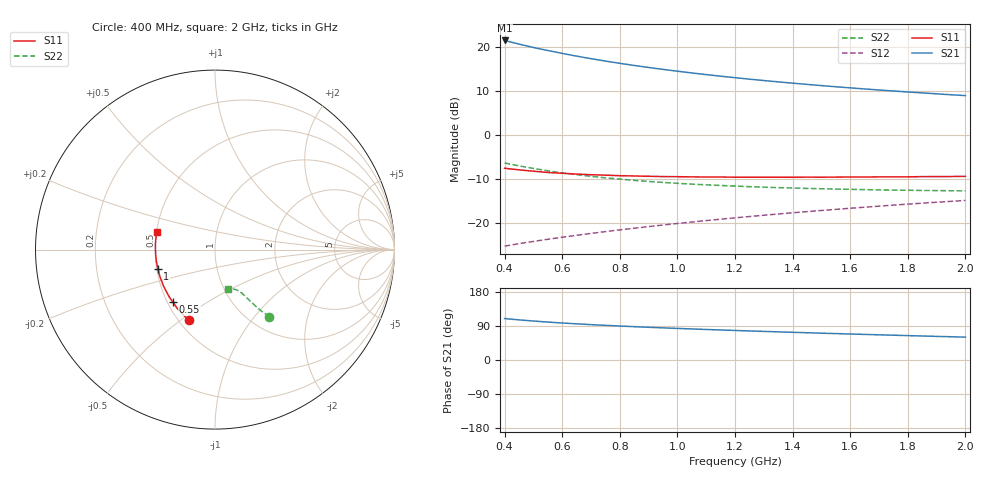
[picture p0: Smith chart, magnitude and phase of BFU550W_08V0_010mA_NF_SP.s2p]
! Filename:  P:\Prog\Test\Noise\ATS_data\Testdata_Net\06 Compressed Noise after Statistics\BFU550W_APM2013_11_D05_08p0V_010mA_NF_CM01_D.sf
! Date/Time: Tue 26/Mar/2013 16:25:24
! BFU550W_APM2013_11_D05_08p0V_1to35mA_NF_CM01_Bias6_R.sf
! Noise Parameter Data File
! BFU550W_APM2013_11_D05_08p0V_1to35mA_NF_CM01
! Date/time: Mon Mar 25 14:39:45 2013
! VAR V_out= 8.000000
! VAR I_out= 9.990000
! VAR V_in= 0.809500
! VAR I_in= 0.099610
! Device data file deembeded for feedlines and parallel
! Original file: \06 Compressed Noise after Statistics\BFU550W_APM2013_11_D05_08p0V_010mA_NF_CM01_R.sf
! Feed-files: PR019V01_070313_Feed1.s2p, PR019V01_070313_Feed2.s2p
! Parallel-file: PR019V01_070313_Par.s2p
# MHz S MA R 50
!  Freq-MHz  S11-mag  S11-arg  S21-mag  S21-arg  S12-mag  S12-arg  S22-mag  S22-arg
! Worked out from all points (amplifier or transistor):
!   37 points, 400 MHz to 2 GHz, reference 50 ohm
!   highest |S21| = 21.4 dB at 400 MHz (marker M1)
!   |S21| within 3 dB of that: start of sweep to 605.1 MHz
!   unconditionally stable (mu >= 1): 1.431 GHz to end of sweep
!   at 500 MHz: K = 0.73, MSG = 22.0 dB, |S12| = -24.1 dB
!   at 1.1 GHz: K = 0.97, MSG = 16.6 dB, |S12| = -19.4 dB
!   at 2 GHz: K = 1.01, MAG = 11.2 dB, |S12| = -14.8 dB
!   lowest NFmin = 0.70 dB at 480 MHz
!   S11 on the Smith chart (normalised r, x): 400 MHz: 0.56, -0.54; 550 MHz: 0.53, -0.36; 1 GHz: 0.51, -0.12; 2 GHz: 0.50, +0.11
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400  0.4195 -110.0  11.79 109.4  0.0548 58.2  0.4809 -50.9
420  0.4118 -113.0  11.34 107.9  0.0563 58.3  0.4666 -51.5
440  0.4053 -115.7  10.92 106.5  0.05775 58.3  0.4527 -52.0
460  0.3993 -118.2  10.53 105.3  0.0592 58.4  0.44 -52.5
500  0.3879 -123.2  9.817 102.8  0.06202 58.6  0.417 -53.4
550  0.3753 -128.6  9.069 100.1  0.06562 59.1  0.3921 -54.2
600  0.3676 -133.6  8.406 97.6  0.0692 59.5  0.371 -54.8
650  0.3599 -138.0  7.827 95.5  0.07279 60.0  0.3544 -55.4
700  0.3541 -142.2  7.324 93.3  0.07646 60.4  0.3393 -56.0
750  0.35 -145.9  6.88 91.5  0.08013 60.9  0.3264 -56.4
800  0.345 -149.5  6.487 89.7  0.08386 61.2  0.3157 -57.0
850  0.3425 -152.9  6.136 87.9  0.08757 61.6  0.3054 -57.2
950  0.3372 -158.6  5.538 84.8  0.09521 62.3  0.2896 -58.1
1000  0.3362 -161.3  5.282 83.4  0.09907 62.5  0.2826 -58.4
1100  0.3334 -166.2  4.834 80.6  0.1069 63.0  0.272 -59.5
1200  0.3319 -170.7  4.461 78.0  0.1149 63.3  0.2632 -60.6
1250  0.3316 -172.9  4.292 76.7  0.1188 63.3  0.2591 -61.0
1350  0.3315 -176.6  3.999 74.3  0.127 63.5  0.2526 -62.2
1500  0.3318 177.9  3.627 70.8  0.1392 63.4  0.2457 -64.2
1650  0.3333 172.9  3.323 67.5  0.1516 63.2  0.24 -66.3
1750  0.3348 170.1  3.152 65.4  0.16 63.0  0.2366 -67.9
2000  0.3394 163.1  2.794 60.3  0.181 62.1  0.2322 -72.4
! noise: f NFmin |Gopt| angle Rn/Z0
400  0.7198  0.1001  155  0.0726
460  0.7224  0.1031  152.1  0.0753
600  0.7451  0.1099  154.5  0.0785
800  0.7865  0.1493  158.9  0.0702
1000  0.8087  0.1575  163.6  0.0716
1200  0.8528  0.1924  167.2  0.0673
1400  0.8746  0.2211  173.9  0.067
1600  0.8819  0.245  178.3  0.0639
1800  0.9404  0.2662  -176.9  0.0638
2000  0.9689  0.2949  -172.9  0.0641
